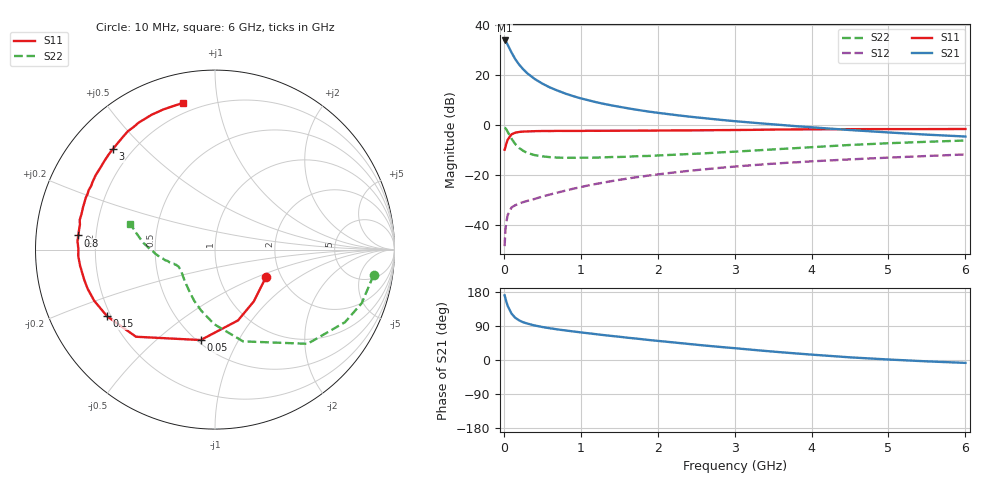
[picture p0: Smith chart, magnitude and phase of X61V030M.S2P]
! SIEMENS Small Signal Semiconductors
! BFP193W
! Si NPN RF Bipolar Junction Transistor in SOT343
! VCE = 1 V  IC = 30 mA
! Common Emitter S-Parameters:  April 1994
# GHz  S  MA  R  50
!  f  S11  S21  S12  S22
! GHz  MAG  ANG  MAG  ANG  MAG  ANG  MAG  ANG
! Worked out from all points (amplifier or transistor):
!   40 points, 10 MHz to 6 GHz, reference 50 ohm
!   highest |S21| = 33.9 dB at 10 MHz (marker M1)
!   |S21| within 3 dB of that: start of sweep to 70.41 MHz
!   unconditionally stable (mu >= 1): 623.3 MHz to end of sweep
!   at 200 MHz: K = 0.50, MSG = 27.7 dB, |S12| = -31.3 dB
!   at 1.5 GHz: K = 1.19, MAG = 12.0 dB, |S12| = -21.9 dB
!   at 6 GHz: K = 1.00, MAG = 3.3 dB, |S12| = -11.7 dB
!   S11 on the Smith chart (normalised r, x): 10 MHz: 1.67, -0.57; 50 MHz: 0.52, -0.71; 150 MHz: 0.19, -0.27; 800 MHz: 0.13, +0.05; 3 GHz: 0.13, +0.40; 6 GHz: 0.15, +0.79
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0.01  0.3228 -28.4  49.31 170.7  0.0038 83.6  0.8949 -9.2
0.02  0.3606 -53.2  48.14 163.3  0.0078 73.9  0.8701 -20.1
0.03  0.4149 -72.0  45.97 155.7  0.0109 69.2  0.8295 -29.2
0.05  0.5102 -99.0  40.38 142.6  0.0159 57.6  0.7359 -45.5
0.1  0.6554 -132.2  28.28 122.3  0.0226 44.2  0.5347 -73.0
0.15  0.7068 -148.3  20.71 111.1  0.0251 39.1  0.4158 -90.6
0.2  0.7307 -157.0  16.12 104.4  0.0271 38.3  0.3479 -102.9
0.25  0.7424 -162.9  13.18 99.8  0.0288 38.4  0.3082 -112.0
0.3  0.7476 -166.9  11.04 96.5  0.0304 40.0  0.2796 -119.4
0.4  0.7568 -173.1  8.4 91.1  0.0334 42.7  0.2513 -129.7
0.5  0.7627 -177.2  6.769 87.1  0.0373 46.4  0.2373 -136.9
0.6  0.7615 179.5  5.656 83.7  0.041 48.7  0.2292 -142.3
0.8  0.7657 174.1  4.273 78.0  0.049 53.0  0.222 -148.7
1.1  0.7717 167.6  3.141 70.5  0.0624 56.2  0.2235 -154.3
1.3  0.7706 163.6  2.662 65.7  0.0712 57.1  0.2271 -156.3
1.6  0.7758 158.2  2.189 59.0  0.085 57.4  0.2332 -158.6
2.2  0.7836 148.0  1.615 46.5  0.1125 55.5  0.2552 -163.4
3  0.7986 135.4  1.2 31.2  0.1484 50.5  0.2945 -170.2
3.2  0.8039 132.2  1.131 27.5  0.1567 49.1  0.3072 -171.9
4.5  0.8301 115.2  0.798 7.0  0.2066 39.4  0.4012 174.6
5.5  0.8326 106.6  0.645 -3.6  0.2413 32.7  0.4642 166.3
6  0.8365 102.3  0.592 -7.6  0.2595 29.6  0.4923 163.0
